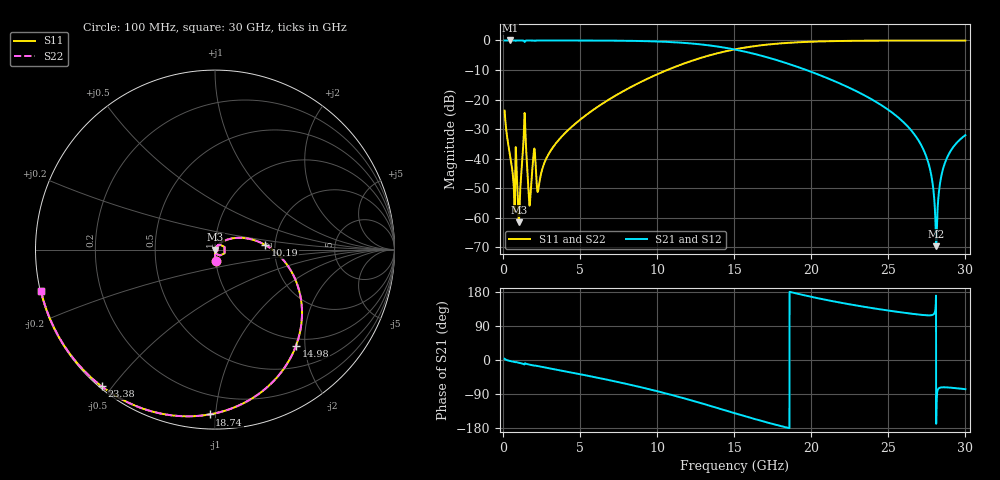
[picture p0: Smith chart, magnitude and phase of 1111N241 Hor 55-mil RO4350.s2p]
# GHz S MA R 50
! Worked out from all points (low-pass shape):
!   3201 points, 100 MHz to 30 GHz, reference 50 ohm
!   highest |S21| = 0.00 dB at 445.7 MHz (marker M1); lowest = -69.6 dB at 28.1 GHz (marker M2)
!   |S21| within 3 dB of the highest: start of sweep to 14.97 GHz
!   lowest |S11| = -61.6 dB at 1.025 GHz (marker M3), VSWR 1.00, Z = 50.1 - j0.00151 ohm
!   |S11| at or under -10 dB: start of sweep to 10.65 GHz
!   |S22| runs from -61.6 to 0.0 dB; largest |S21 - S12| = 2.8e-11
!   S11 on the Smith chart (normalised r, x): 100 MHz: 1.00, -0.13; 10.19 GHz: 1.77, +0.10; 14.98 GHz: 0.86, -1.82; 18.74 GHz: 0.08, -0.96; 23.38 GHz: 0.01, -0.47; 30 GHz: 0.00, -0.12
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0.1  0.06516 -86.8  0.9976 3.0  0.9976 3.0  0.06516 -86.8
0.4457187  0.01174 -90.7  0.9995 -2.5  0.9995 -2.5  0.01174 -90.7
1.025031  0.0008332 -1.0  0.9991 -7.3  0.9991 -7.3  0.0008332 -1.0
1.380094  0.04773 29.7  0.9635 -11.7  0.9635 -11.7  0.04773 29.7
1.735156  0.001678 4.8  0.9982 -12.4  0.9982 -12.4  0.001678 4.8
1.987437  0.01255 32.0  0.9911 -14.7  0.9911 -14.7  0.01255 32.0
2.314469  0.003342 39.4  0.9979 -16.6  0.9979 -16.6  0.003342 39.4
3.127375  0.01417 62.9  0.9985 -22.9  0.9985 -22.9  0.01417 62.9
5.089563  0.04766 50.4  0.9972 -38.3  0.9972 -38.3  0.04766 50.4
10.06978  0.2724 6.5  0.9589 -83.0  0.9589 -83.0  0.2724 6.5
10.19125  0.2812 5.3  0.9563 -84.3  0.9563 -84.3  0.2812 5.3
14.98459  0.7017 -50.1  0.7065 -139.8  0.7065 -139.8  0.7017 -50.1
15.05  0.7071 -50.9  0.7011 -140.6  0.7011 -140.6  0.7071 -50.9
18.74078  0.9188 -91.9  0.3851 178.4  0.3851 178.4  0.9188 -91.9
20.03956  0.9528 -103.9  0.2917 166.4  0.2917 166.4  0.9528 -103.9
23.37528  0.9895 -129.7  0.1207 140.8  0.1207 140.8  0.9895 -129.7
25.01978  0.9947 -140.2  0.06644 130.4  0.06644 130.4  0.9947 -140.2
27.29031  0.9968 -153.0  0.01401 118.6  0.01401 118.6  0.9968 -153.0
27.7575  0.9969 -155.5  0.005737 118.0  0.005737 118.0  0.9969 -155.5
28.10322  0.9969 -157.3  0.0003313 -168.3  0.0003313 -168.3  0.9969 -157.3
28.70122  0.9969 -160.3  0.008882 -72.1  0.008882 -72.1  0.9969 -160.3
30  0.9966 -166.5  0.02501 -77.0  0.02501 -77.0  0.9966 -166.5
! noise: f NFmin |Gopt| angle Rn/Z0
0.1  0.0006418  0.7259  0.9094  0.0004652
3.417  0.008471  0.4232  23.74  0.002321
6.743  0.01415  0.3675  43.44  0.003142
10.06  0.02141  0.3962  59.51  0.004559
13.39  0.03233  0.4813  74.63  0.007202
16.7  0.0519  0.6136  91.79  0.01283
20.03  0.09478  0.7629  111.4  0.02675
23.35  0.2171  0.8885  131.4  0.07306
26.67  1.003  0.9742  149.9  0.603
30  1.074  0.9751  166.4  0.1398
